| IBIS file stm32l0_51_52_53_62_63_lqfp48.ibs
| Created by s2ibis version 1.1 (customized version)
| North Carolina State University, ERL, 2006
[IBIS ver] 4.2
[File name] stm32l0_51_52_53_62_63_lqfp48.ibs
[File Rev] 1.0
[Date]  15-10-2014
[Source] Data Created at STMicroelectronics
[Notes]  File originated from ELDO simulations.
[Disclaimer]  This information is for modeling purpose only and is
   not guaranted. The information is subject to change without
   notice.
[Copyright] Copyright 2016 STMicroelectronics Inc.
|   Component stm32l0_51_52_53_62_63_lqfp48
[Component] stm32l0_51_52_53_62_63_lqfp48
[Manufacturer] STMicroelectronics
[Package]
| variable   typ   min   max
R_pkg   0.0   0.0   0.0
L_pkg   0.0H   0.0H   0.0H
C_pkg   0.0F   0.0F   0.0F
[Pin]  signal_name   model_name   R_pin   L_pin   C_pin
1 VLCD POWER 0.053 3.42534E-09 9.041E-14
2 PC13 io8p_wsudq_ls_ft_v33 0.048377332 2.91404E-09 6.443E-14
3 PC14-OSC32_IN io8p_wsudq_ls_ft_v33 0.044678997 2.50442E-09 4.365E-14
4 PC15-OSC32_OUT io8p_sudq_ls_tc_esdft 0.041905328 2.19704E-09 2.807E-14
5 PH0-OSC_IN io8p_sudq_ls_tc_esdft 0.040056325 1.9919E-09 1.769E-14
6 PH1-OSC_OUT io8p_sudq_ls_tc_esdft 0.03913 1.89021E-09 1.24625E-14
7 NRST ioreset_tc_v33_esdft 0.03913 1.89021E-09 1.24625E-14
8 VSSA GND 0.040057312 1.98992E-09 1.775E-14
9 VDDA POWER 0.041906973 2.19374E-09 2.817E-14
10 PA0 io8p_wsudq_ls_ft_v33 0.0446813 2.4998E-09 4.379E-14
11 PA1 io8p_wsudq_lcd4_ls_ft 0.048380293 2.9081E-09 6.461E-14
12 PA2 io8p_wsudq_lcd4_ls_ft 0.053 3.42534E-09 9.041E-14
13 PA3 io8p_wsudq_lcd4_ls_ft 0.053 3.42534E-09 9.041E-14
14 PA4 io8p_wsudq_i2cin_ls_ft 0.048377332 2.91404E-09 6.443E-14
15 PA5 io8p_wsudq_i2cin_ls_ft 0.044678997 2.50442E-09 4.365E-14
16 PA6 io8p_wsudq_lcd4_ls_ft 0.041905328 2.19704E-09 2.807E-14
17 PA7 io8p_wsudq_lcd4_ls_ft 0.040056325 1.9919E-09 1.769E-14
18 PB0 io8p_wsudq_lcd4_ls_ft 0.03913 1.89021E-09 1.24625E-14
19 PB1 io8p_wsudq_lcd4_ls_ft 0.03913 1.89021E-09 1.24625E-14
20 PB2 io8p_wsudq_lcd4_ls_ft 0.040057312 1.98992E-09 1.775E-14
21 PB10 io8p_sudq_lcd4_i2cin_ls_ft 0.041906973 2.19374E-09 2.817E-14
22 PB11 io8p_sudq_lcd4_i2cin_ls_ft 0.0446813 2.4998E-09 4.379E-14
23 VSS GND 0.048380293 2.9081E-09 6.461E-14
24 VDD POWER 0.053 3.42534E-09 9.041E-14
25 PB12 io8p_wsudq_lcd4_ls_ft 0.053 3.42534E-09 9.041E-14
26 PB13 io8p_sudq_lcd4_i2cin_ls_ft 0.048377332 2.91404E-09 6.443E-14
27 PB14 io8p_sudq_lcd4_i2cin_ls_ft 0.044678997 2.50442E-09 4.365E-14
28 PB15 io8p_wsudq_lcd4_ls_ft 0.041905328 2.19704E-09 2.807E-14
29 PA8 io8p_wsudq_lcd4_ls_ft 0.040056325 1.9919E-09 1.769E-14
30 PA9 io8p_wsudq_lcd4_ls_ft 0.03913 1.89021E-09 1.24625E-14
31 PA10 io8p_wsudq_lcd4_ls_ft 0.03913 1.89021E-09 1.24625E-14
32 PA11 io8usb_ls_ft 0.040057312 1.98992E-09 1.775E-14
33 PA12 io8usb_ls_ft 0.041906973 2.19374E-09 2.817E-14
34 PA13 io8p_sudq_ls_ft 0.0446813 2.4998E-09 4.379E-14
35 VSS GND 0.048380293 2.9081E-09 6.461E-14
36 VDD_USB POWER 0.053 3.42534E-09 9.041E-14
37 PA14 io8p_sudq_ls_ft 0.053 3.42534E-09 9.041E-14
38 PA15 io8p_wsudq_lcd4_ls_ft 0.048377332 2.91404E-09 6.443E-14
39 PB3 io8p_wsudq_lcd4_ls_ft 0.044678997 2.50442E-09 4.365E-14
40 PB4 io8p_wsudq_lcd4_ls_ft 0.041905328 2.19704E-09 2.807E-14
41 PB5 io8p_wsudq_lcd4_ls_ft 0.040056325 1.9919E-09 1.769E-14
42 PB6 io8p_wsudq_i2cin_ls_ft 0.03913 1.89021E-09 1.24625E-14
43 PB7 io8p_wsudq_i2cin_ls_ft 0.03913 1.89021E-09 1.24625E-14
44 BOOT0 vpp_test_hv 0.040057312 1.98992E-09 1.775E-14
45 PB8 io8p_sudq_lcd4_i2cin_ls_ft 0.041906973 2.19374E-09 2.817E-14
46 PB9 io8p_sudq_lcd4_i2cin_ls_ft 0.0446813 2.4998E-09 4.379E-14
47 VSS GND 0.048380293 2.9081E-09 6.461E-14
48 VDD POWER 0.053 3.42534E-09 9.041E-14
[Model Selector] io8p_sudq_ls_ft
io8p00_sudq_ls_ft_pd_lv  "SPEED00 1P8V, PD=40kOhm"
io8p00_sudq_ls_ft_pu_lv  "SPEED00 1P8V, PU=40kOhm"
io8p00_sudq_ls_ft_lv  "SPEED00 1P8V"
io8p01_sudq_ls_ft_pd_lv  "SPEED01 1P8V, PD=40kOhm"
io8p01_sudq_ls_ft_pu_lv  "SPEED01 1P8V, PU=40kOhm"
io8p01_sudq_ls_ft_lv  "SPEED01 1P8V"
io8p10_sudq_ls_ft_pd_lv  "SPEED10 1P8V, PD=40kOhm"
io8p10_sudq_ls_ft_pu_lv  "SPEED10 1P8V, PU=40kOhm"
io8p10_sudq_ls_ft_lv  "SPEED10 1P8V"
io8p11_sudq_ls_ft_pd_lv  "SPEED11 1P8V, PD=40kOhm"
io8p11_sudq_ls_ft_pu_lv  "SPEED11 1P8V, PU=40kOhm"
io8p11_sudq_ls_ft_lv  "SPEED11 1P8V"
io8p00_sudq_ls_ft_pd  "SPEED00, PD=40kOhm"
io8p00_sudq_ls_ft_pu  "SPEED00, PU=40kOhm"
io8p00_sudq_ls_ft  "SPEED00"
io8p01_sudq_ls_ft_pd  "SPEED01, PD=40kOhm"
io8p01_sudq_ls_ft_pu  "SPEED01, PU=40kOhm"
io8p01_sudq_ls_ft  "SPEED01"
io8p10_sudq_ls_ft_pd  "SPEED10, PD=40kOhm"
io8p10_sudq_ls_ft_pu  "SPEED10, PU=40kOhm"
io8p10_sudq_ls_ft  "SPEED10"
io8p11_sudq_ls_ft_pd  "SPEED11, PD=40kOhm"
io8p11_sudq_ls_ft_pu  "SPEED11, PU=40kOhm"
io8p11_sudq_ls_ft  "SPEED11"
[Model Selector] io8p_sudq_ls_tc_esdft
io8p00_sudq_ls_tc_esdft_pd_lv  "SPEED00 1P8V, PD=40kOhm"
io8p00_sudq_ls_tc_esdft_pu_lv  "SPEED00 1P8V, PU=40kOhm"
io8p00_sudq_ls_tc_esdft_lv  "SPEED00 1P8V"
io8p01_sudq_ls_tc_esdft_pd_lv  "SPEED01 1P8V, PD=40kOhm"
io8p01_sudq_ls_tc_esdft_pu_lv  "SPEED01 1P8V, PU=40kOhm"
io8p01_sudq_ls_tc_esdft_lv  "SPEED01 1P8V"
io8p10_sudq_ls_tc_esdft_pd_lv  "SPEED10 1P8V, PD=40kOhm"
io8p10_sudq_ls_tc_esdft_pu_lv  "SPEED10 1P8V, PU=40kOhm"
io8p10_sudq_ls_tc_esdft_lv  "SPEED10 1P8V"
io8p11_sudq_ls_tc_esdft_pd_lv  "SPEED11 1P8V, PD=40kOhm"
io8p11_sudq_ls_tc_esdft_pu_lv  "SPEED11 1P8V, PU=40kOhm"
io8p11_sudq_ls_tc_esdft_lv  "SPEED11 1P8V"
io8p00_sudq_ls_tc_esdft_pd  "SPEED00, PD=40kOhm"
io8p00_sudq_ls_tc_esdft_pu  "SPEED00, PU=40kOhm"
io8p00_sudq_ls_tc_esdft  "SPEED00"
io8p01_sudq_ls_tc_esdft_pd  "SPEED01, PD=40kOhm"
io8p01_sudq_ls_tc_esdft_pu  "SPEED01, PU=40kOhm"
io8p01_sudq_ls_tc_esdft  "SPEED01"
io8p10_sudq_ls_tc_esdft_pd  "SPEED10, PD=40kOhm"
io8p10_sudq_ls_tc_esdft_pu  "SPEED10, PU=40kOhm"
io8p10_sudq_ls_tc_esdft  "SPEED10"
io8p11_sudq_ls_tc_esdft_pd  "SPEED11, PD=40kOhm"
io8p11_sudq_ls_tc_esdft_pu  "SPEED11, PU=40kOhm"
io8p11_sudq_ls_tc_esdft  "SPEED11"
[Model Selector] io8p_wsudq_i2cin_ls_ft
io8p00_wsudq_i2cin_ls_ft_pd_lv  "SPEED00 1P8V, PD=40kOhm"
io8p00_wsudq_i2cin_ls_ft_pu_lv  "SPEED00 1P8V, PU=40kOhm"
io8p00_wsudq_i2cin_ls_ft_lv  "SPEED00 1P8V"
io8p01_wsudq_i2cin_ls_ft_pd_lv  "SPEED01 1P8V, PD=40kOhm"
io8p01_wsudq_i2cin_ls_ft_pu_lv  "SPEED01 1P8V, PU=40kOhm"
io8p01_wsudq_i2cin_ls_ft_lv  "SPEED01 1P8V"
io8p10_wsudq_i2cin_ls_ft_pd_lv  "SPEED10 1P8V, PD=40kOhm"
io8p10_wsudq_i2cin_ls_ft_pu_lv  "SPEED10 1P8V, PU=40kOhm"
io8p10_wsudq_i2cin_ls_ft_lv  "SPEED10 1P8V"
io8p11_wsudq_i2cin_ls_ft_pd_lv  "SPEED11 1P8V, PD=40kOhm"
io8p11_wsudq_i2cin_ls_ft_pu_lv  "SPEED11 1P8V, PU=40kOhm"
io8p11_wsudq_i2cin_ls_ft_lv  "SPEED11 1P8V"
io8p00_wsudq_i2cin_ls_ft_pd  "SPEED00, PD=40kOhm"
io8p00_wsudq_i2cin_ls_ft_pu  "SPEED00, PU=40kOhm"
io8p00_wsudq_i2cin_ls_ft  "SPEED00"
io8p01_wsudq_i2cin_ls_ft_pd  "SPEED01, PD=40kOhm"
io8p01_wsudq_i2cin_ls_ft_pu  "SPEED01, PU=40kOhm"
io8p01_wsudq_i2cin_ls_ft  "SPEED01"
io8p10_wsudq_i2cin_ls_ft_pd  "SPEED10, PD=40kOhm"
io8p10_wsudq_i2cin_ls_ft_pu  "SPEED10, PU=40kOhm"
io8p10_wsudq_i2cin_ls_ft  "SPEED10"
io8p11_wsudq_i2cin_ls_ft_pd  "SPEED11, PD=40kOhm"
io8p11_wsudq_i2cin_ls_ft_pu  "SPEED11, PU=40kOhm"
io8p11_wsudq_i2cin_ls_ft  "SPEED11"
[Model Selector] io8p_wsudq_lcd4_ls_ft
io8p00_wsudq_lcd4_ls_ft_pd_lv  "SPEED00 1P8V, PD=40kOhm"
io8p00_wsudq_lcd4_ls_ft_pu_lv  "SPEED00 1P8V, PU=40kOhm"
io8p00_wsudq_lcd4_ls_ft_lv  "SPEED00 1P8V"
io8p01_wsudq_lcd4_ls_ft_pd_lv  "SPEED01 1P8V, PD=40kOhm"
io8p01_wsudq_lcd4_ls_ft_pu_lv  "SPEED01 1P8V, PU=40kOhm"
io8p01_wsudq_lcd4_ls_ft_lv  "SPEED01 1P8V"
io8p10_wsudq_lcd4_ls_ft_pd_lv  "SPEED10 1P8V, PD=40kOhm"
io8p10_wsudq_lcd4_ls_ft_pu_lv  "SPEED10 1P8V, PU=40kOhm"
io8p10_wsudq_lcd4_ls_ft_lv  "SPEED10 1P8V"
io8p11_wsudq_lcd4_ls_ft_pd_lv  "SPEED11 1P8V, PD=40kOhm"
io8p11_wsudq_lcd4_ls_ft_pu_lv  "SPEED11 1P8V, PU=40kOhm"
io8p11_wsudq_lcd4_ls_ft_lv  "SPEED11 1P8V"
io8p00_wsudq_lcd4_ls_ft_pd  "SPEED00, PD=40kOhm"
io8p00_wsudq_lcd4_ls_ft_pu  "SPEED00, PU=40kOhm"
io8p00_wsudq_lcd4_ls_ft  "SPEED00"
io8p01_wsudq_lcd4_ls_ft_pd  "SPEED01, PD=40kOhm"
io8p01_wsudq_lcd4_ls_ft_pu  "SPEED01, PU=40kOhm"
io8p01_wsudq_lcd4_ls_ft  "SPEED01"
io8p10_wsudq_lcd4_ls_ft_pd  "SPEED10, PD=40kOhm"
io8p10_wsudq_lcd4_ls_ft_pu  "SPEED10, PU=40kOhm"
io8p10_wsudq_lcd4_ls_ft  "SPEED10"
io8p11_wsudq_lcd4_ls_ft_pd  "SPEED11, PD=40kOhm"
io8p11_wsudq_lcd4_ls_ft_pu  "SPEED11, PU=40kOhm"
io8p11_wsudq_lcd4_ls_ft  "SPEED11"
[Model Selector] io8p_wsudq_ls_ft_v33
io8p00_wsudq_ls_ft_v33_pd_lv  "SPEED00 1P8V, PD=40kOhm"
io8p00_wsudq_ls_ft_v33_pu_lv  "SPEED00 1P8V, PU=40kOhm"
io8p00_wsudq_ls_ft_v33_lv  "SPEED00 1P8V"
io8p01_wsudq_ls_ft_v33_pd_lv  "SPEED01 1P8V, PD=40kOhm"
io8p01_wsudq_ls_ft_v33_pu_lv  "SPEED01 1P8V, PU=40kOhm"
io8p01_wsudq_ls_ft_v33_lv  "SPEED01 1P8V"
io8p10_wsudq_ls_ft_v33_pd_lv  "SPEED10 1P8V, PD=40kOhm"
io8p10_wsudq_ls_ft_v33_pu_lv  "SPEED10 1P8V, PU=40kOhm"
io8p10_wsudq_ls_ft_v33_lv  "SPEED10 1P8V"
io8p11_wsudq_ls_ft_v33_pd_lv  "SPEED11 1P8V, PD=40kOhm"
io8p11_wsudq_ls_ft_v33_pu_lv  "SPEED11 1P8V, PU=40kOhm"
io8p11_wsudq_ls_ft_v33_lv  "SPEED11 1P8V"
io8p00_wsudq_ls_ft_v33_pd  "SPEED00, PD=40kOhm"
io8p00_wsudq_ls_ft_v33_pu  "SPEED00, PU=40kOhm"
io8p00_wsudq_ls_ft_v33  "SPEED00"
io8p01_wsudq_ls_ft_v33_pd  "SPEED01, PD=40kOhm"
io8p01_wsudq_ls_ft_v33_pu  "SPEED01, PU=40kOhm"
io8p01_wsudq_ls_ft_v33  "SPEED01"
io8p10_wsudq_ls_ft_v33_pd  "SPEED10, PD=40kOhm"
io8p10_wsudq_ls_ft_v33_pu  "SPEED10, PU=40kOhm"
io8p10_wsudq_ls_ft_v33  "SPEED10"
io8p11_wsudq_ls_ft_v33_pd  "SPEED11, PD=40kOhm"
io8p11_wsudq_ls_ft_v33_pu  "SPEED11, PU=40kOhm"
io8p11_wsudq_ls_ft_v33  "SPEED11"
[Model Selector] ioreset_tc_v33_esdft
ioreset_tc_v33_esdft_pu_lv  "IORESET 1P65V + PU=40kOhm"
ioreset_tc_v33_esdft_nopu_lv  "IORESET 1P65V"
ioreset_tc_v33_esdft_pu  "IORESET + PU=40kOhm"
ioreset_tc_v33_esdft_nopu  "IORESET"
[Model Selector] vpp_test_hv
vpp_test_hv_2p4  "Input Buffer 1P65V"
vpp_test_hv_3p3  "Input Buffer"
[Model Selector] io8usb_ls_ft
io8usb_ls_ft_dpdn_pu  "HS USB DP/DN IO + PU=1.2kOhm"
io8usb_ls_ft_dpdn  "HS USB DP/DN IO"
io8p00_ls_ft_pd_lv  "SPEED00 1P8V, PD=40kOhm"
io8p00_ls_ft_pu_lv  "SPEED00 1P8V, PU=40kOhm"
io8p00_ls_ft_lv  "SPEED00 1P8V"
io8p01_ls_ft_pd_lv  "SPEED01 1P8V, PD=40kOhm"
io8p01_ls_ft_pu_lv  "SPEED01 1P8V, PU=40kOhm"
io8p01_ls_ft_lv  "SPEED01 1P8V"
io8p10_ls_ft_pd_lv  "SPEED10 1P8V, PD=40kOhm"
io8p10_ls_ft_pu_lv  "SPEED10 1P8V, PU=40kOhm"
io8p10_ls_ft_lv  "SPEED10 1P8V"
io8p11_ls_ft_pd_lv  "SPEED11 1P8V, PD=40kOhm"
io8p11_ls_ft_pu_lv  "SPEED11 1P8V, PU=40kOhm"
io8p11_ls_ft_lv  "SPEED11 1P8V"
io8p00_ls_ft_pd  "SPEED00, PD=40kOhm"
io8p00_ls_ft_pu  "SPEED00, PU=40kOhm"
io8p00_ls_ft  "SPEED00"
io8p01_ls_ft_pd  "SPEED01, PD=40kOhm"
io8p01_ls_ft_pu  "SPEED01, PU=40kOhm"
io8p01_ls_ft  "SPEED01"
io8p10_ls_ft_pd  "SPEED10, PD=40kOhm"
io8p10_ls_ft_pu  "SPEED10, PU=40kOhm"
io8p10_ls_ft  "SPEED10"
io8p11_ls_ft_pd  "SPEED11, PD=40kOhm"
io8p11_ls_ft_pu  "SPEED11, PU=40kOhm"
io8p11_ls_ft  "SPEED11"
[Model Selector] io8p_sudq_lcd4_i2cin_ls_ft
io8p00_sudq_lcd4_i2cin_ls_ft_pd_lv  "SPEED00 1P8V, PD=40kOhm"
io8p00_sudq_lcd4_i2cin_ls_ft_pu_lv  "SPEED00 1P8V, PU=40kOhm"
io8p00_sudq_lcd4_i2cin_ls_ft_lv  "SPEED00 1P8V"
io8p01_sudq_lcd4_i2cin_ls_ft_pd_lv  "SPEED01 1P8V, PD=40kOhm"
io8p01_sudq_lcd4_i2cin_ls_ft_pu_lv  "SPEED01 1P8V, PU=40kOhm"
io8p01_sudq_lcd4_i2cin_ls_ft_lv  "SPEED01 1P8V"
io8p10_sudq_lcd4_i2cin_ls_ft_pd_lv  "SPEED10 1P8V, PD=40kOhm"
io8p10_sudq_lcd4_i2cin_ls_ft_pu_lv  "SPEED10 1P8V, PU=40kOhm"
io8p10_sudq_lcd4_i2cin_ls_ft_lv  "SPEED10 1P8V"
io8p11_sudq_lcd4_i2cin_ls_ft_pd_lv  "SPEED11 1P8V, PD=40kOhm"
io8p11_sudq_lcd4_i2cin_ls_ft_pu_lv  "SPEED11 1P8V, PU=40kOhm"
io8p11_sudq_lcd4_i2cin_ls_ft_lv  "SPEED11 1P8V"
io8p00_sudq_lcd4_i2cin_ls_ft_pd  "SPEED00, PD=40kOhm"
io8p00_sudq_lcd4_i2cin_ls_ft_pu  "SPEED00, PU=40kOhm"
io8p00_sudq_lcd4_i2cin_ls_ft  "SPEED00"
io8p01_sudq_lcd4_i2cin_ls_ft_pd  "SPEED01, PD=40kOhm"
io8p01_sudq_lcd4_i2cin_ls_ft_pu  "SPEED01, PU=40kOhm"
io8p01_sudq_lcd4_i2cin_ls_ft  "SPEED01"
io8p10_sudq_lcd4_i2cin_ls_ft_pd  "SPEED10, PD=40kOhm"
io8p10_sudq_lcd4_i2cin_ls_ft_pu  "SPEED10, PU=40kOhm"
io8p10_sudq_lcd4_i2cin_ls_ft  "SPEED10"
io8p11_sudq_lcd4_i2cin_ls_ft_pd  "SPEED11, PD=40kOhm"
io8p11_sudq_lcd4_i2cin_ls_ft_pu  "SPEED11, PU=40kOhm"
io8p11_sudq_lcd4_i2cin_ls_ft  "SPEED11"
| Models and submodels in the file (176): io8p00_sudq_ls_ft_pd_lv (I/O), io8p00_sudq_ls_ft_pu_lv (I/O), io8p00_sudq_ls_ft_lv (I/O), io8p01_sudq_ls_ft_pd_lv (I/O), io8p01_sudq_ls_ft_pu_lv (I/O), io8p01_sudq_ls_ft_lv (I/O), io8p10_sudq_ls_ft_pd_lv (I/O), io8p10_sudq_ls_ft_pu_lv (I/O), io8p10_sudq_ls_ft_lv (I/O), io8p11_sudq_ls_ft_pd_lv (I/O), io8p11_sudq_ls_ft_pu_lv (I/O), io8p11_sudq_ls_ft_lv (I/O), io8p00_sudq_ls_ft_pd (I/O), io8p00_sudq_ls_ft_pu (I/O), io8p00_sudq_ls_ft (I/O), io8p01_sudq_ls_ft_pd (I/O), io8p01_sudq_ls_ft_pu (I/O), io8p01_sudq_ls_ft (I/O), io8p10_sudq_ls_ft_pd (I/O), io8p10_sudq_ls_ft_pu (I/O), io8p10_sudq_ls_ft (I/O), io8p11_sudq_ls_ft_pd (I/O), io8p11_sudq_ls_ft_pu (I/O), io8p11_sudq_ls_ft (I/O), io8p00_sudq_ls_tc_esdft_pd_lv (I/O), io8p00_sudq_ls_tc_esdft_pu_lv (I/O), io8p00_sudq_ls_tc_esdft_lv (I/O), io8p01_sudq_ls_tc_esdft_pd_lv (I/O), io8p01_sudq_ls_tc_esdft_pu_lv (I/O), io8p01_sudq_ls_tc_esdft_lv (I/O), io8p10_sudq_ls_tc_esdft_pd_lv (I/O), io8p10_sudq_ls_tc_esdft_pu_lv (I/O), io8p10_sudq_ls_tc_esdft_lv (I/O), io8p11_sudq_ls_tc_esdft_pd_lv (I/O), io8p11_sudq_ls_tc_esdft_pu_lv (I/O), io8p11_sudq_ls_tc_esdft_lv (I/O), io8p00_sudq_ls_tc_esdft_pd (I/O), io8p00_sudq_ls_tc_esdft_pu (I/O), io8p00_sudq_ls_tc_esdft (I/O), io8p01_sudq_ls_tc_esdft_pd (I/O), io8p01_sudq_ls_tc_esdft_pu (I/O), io8p01_sudq_ls_tc_esdft (I/O), io8p10_sudq_ls_tc_esdft_pd (I/O), io8p10_sudq_ls_tc_esdft_pu (I/O), io8p10_sudq_ls_tc_esdft (I/O), io8p11_sudq_ls_tc_esdft_pd (I/O), io8p11_sudq_ls_tc_esdft_pu (I/O), io8p11_sudq_ls_tc_esdft (I/O), io8p00_wsudq_i2cin_ls_ft_pd_lv (I/O), io8p00_wsudq_i2cin_ls_ft_pu_lv (I/O), io8p00_wsudq_i2cin_ls_ft_lv (I/O), io8p01_wsudq_i2cin_ls_ft_pd_lv (I/O), io8p01_wsudq_i2cin_ls_ft_pu_lv (I/O), io8p01_wsudq_i2cin_ls_ft_lv (I/O), io8p10_wsudq_i2cin_ls_ft_pd_lv (I/O), io8p10_wsudq_i2cin_ls_ft_pu_lv (I/O), io8p10_wsudq_i2cin_ls_ft_lv (I/O), io8p11_wsudq_i2cin_ls_ft_pd_lv (I/O), io8p11_wsudq_i2cin_ls_ft_pu_lv (I/O), io8p11_wsudq_i2cin_ls_ft_lv (I/O), io8p00_wsudq_i2cin_ls_ft_pd (I/O), io8p00_wsudq_i2cin_ls_ft_pu (I/O), io8p00_wsudq_i2cin_ls_ft (I/O), io8p01_wsudq_i2cin_ls_ft_pd (I/O), io8p01_wsudq_i2cin_ls_ft_pu (I/O), io8p01_wsudq_i2cin_ls_ft (I/O), io8p10_wsudq_i2cin_ls_ft_pd (I/O), io8p10_wsudq_i2cin_ls_ft_pu (I/O), io8p10_wsudq_i2cin_ls_ft (I/O), io8p11_wsudq_i2cin_ls_ft_pd (I/O), io8p11_wsudq_i2cin_ls_ft_pu (I/O), io8p11_wsudq_i2cin_ls_ft (I/O), io8p00_wsudq_lcd4_ls_ft_pd_lv (I/O), io8p00_wsudq_lcd4_ls_ft_pu_lv (I/O), io8p00_wsudq_lcd4_ls_ft_lv (I/O), io8p01_wsudq_lcd4_ls_ft_pd_lv (I/O), io8p01_wsudq_lcd4_ls_ft_pu_lv (I/O), io8p01_wsudq_lcd4_ls_ft_lv (I/O), io8p10_wsudq_lcd4_ls_ft_pd_lv (I/O), io8p10_wsudq_lcd4_ls_ft_pu_lv (I/O)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
